// TwinCAT 3 PLC project TC_Sample
// ProgramVersion: 3.1.4023.0
// libraries:
//   Tc2_ControllerToolbox, * (Beckhoff Automation GmbH)
//   Tc2_Standard, * (Beckhoff Automation GmbH)
//   Tc2_System, * (Beckhoff Automation GmbH)
//   Tc2_TempController, * (Beckhoff Automation GmbH)
//   Tc3_Module, * (Beckhoff Automation GmbH)
//   VisuDialogs, * (System)
//   VisuSymbols,3.5.10.0,System
// project tree:
//   / GlobalTextList.TcGTLO, PlcTask.TcTTO, Visualization Manager.TcVMO
//   GVLs/ Scope_Variables.TcGVL
//   POUs/Controller/ Controller_v2.TcPOU
//   POUs/ MAIN.TcPOU
//   VISUs/ Visualization.TcVIS
// real-time tasks:
//   TASK PlcTask: cycle T#10ms, priority 20, ADS port 350
// I/O:
//   DEVICE Device 1 (EtherCAT), AmsNetId 5.47.60.12.2.1
//     Term 1 (EK1200) [EK1200-5000 EtherCAT Power supply (2A E-Bus)]
//       Term 2 (EL3204) [EL3204 4Ch. Ana. Input PT100 (RTD)]
//       Term 3 (EL2004) [EL2004 4Ch. Dig. Output 24V, 0.5A]
//       Term 4 (EL9011) [EL9011 End Terminal]
// variable links:
//   TC_Sample/TC_Sample Instance <-> Device 1 (EtherCAT)/Term 1 (EK1200)/Term 2 (EL3204)
//     PlcTask Inputs/Controller_v2.iTempre <-> RTD Inputs Channel 1/Value
//   TC_Sample/TC_Sample Instance <-> Device 1 (EtherCAT)/Term 1 (EK1200)/Term 3 (EL2004)
//     PlcTask Outputs/Controller_v2.bYPWMPos <-> Channel 1/Output

CONFIGURATION TC_Sample
    RESOURCE PLC ON TwinCAT3
        TASK PlcTask(INTERVAL := T#10ms, PRIORITY := 20);
        PROGRAM MAIN WITH PlcTask : MAIN;
    END_RESOURCE
END_CONFIGURATION

// ---- GVLs/Scope_Variables.TcGVL
VAR_GLOBAL
	fX_Scope	: LREAL;
	fY_Scope	: LREAL;
	fW_Scope	: LREAL;
END_VAR

// ---- POUs/MAIN.TcPOU
PROGRAM MAIN

VAR	
(* 选择功能块，温度控制库有两个功能块版本 V1和 V2 ，系统通过默认选择 V1，V1为旧版本，已被淘汰 *)
	nSelectController	: UINT := 1;	
	
(* 激活系统触发条件 *)	
	bStart				: BOOL;			
END_VAR

(* 调用功能块V2，需将nSelectController从1切换为2 *)
IF bStart THEN
	       	nSelectController:= 2  ;   
			Controller_v2();		
END_IF;

END_PROGRAM

// ---- POUs/Controller/Controller_v2.TcPOU
PROGRAM Controller_v2

VAR
	
		eCTRL_Mode 				: E_CTRL_MODE := eCTRL_MODE_Tune; 	(*控制模式*)
		bSelSetpoint			: BOOL	:= FALSE;
		
			iTempre AT %I*:INT;                                  (* 传输回未被转换的温度值 *)
			ftemp:LREAL;                                         (* 被转换的实际温度值 *)
		
		fW						: LREAL;						(* 设定值 *)
		fW1						: LREAL := 65.0;				(* 主设定值*)
		fW2						: LREAL := 45.0;				(* 辅助设定值*)		
		fY						: LREAL;						(* 模拟量输出中间变量 *)
		fX						: LREAL;						(* 设备真实的温度值 *)
		bYPWMPos				AT %Q*: BOOL;                   (* PWM输出，加热 *)
		bYPWMNeg				AT %Q*: BOOL;                   (* PWM输出，冷却 *)
		
		bNoise					: BOOL;                         (* 系统中是否存在错误 *)
		bError 					: BOOL;                         (* 存在错误的话，会生成一个错误代码 *)
		eErrorId 				: E_CTRL_ErrorCodes;
		
		stControllerParameter	: ST_CTRL_TempCtrlParameter := (		
		
		(*内部结构体参数 *)
		iMode					:= 1,											(*运作模式 ： 1=加热, 2=冷却, 3=加热以及冷却 *)
		iReactionOnFailure		:= eCTRL_ReactionOnFailure_StopController,		(*当系统产生错误时，系统反应： 0=关闭系统, 1=手动操作 *)
	
		bSelCtrlParameterSet	:= FALSE,										(* FALSE = 内部pid设定, TRUE = 外部pid设定 *)
	
		dwAlarmSupp				:= 16#0000EFFF,									(* 报警限制值 *)
		tCtrlCycleTime			:= T#500MS,										(* 控制器周期时间 *)
		tTaskCycleTime			:= T#10MS,										(* PLC任务周期时间 *)
		
		(*整定参数*)
		iTuningMode				:= 1,											(* 只加热、只冷却、先加热后冷却、先冷却后加热 *)
	
		tTuneStabilisation		:= T#5S,										(* 等待系统稳定下的时间 *)
	
		fEndTunePercentHeating	:= 80.0,										(* 大于80%，切换成闭环控制 *)
		fYTuneHeating			:= 100.0,										(* 加热协调操作时的阶跃变换 *)
		fYStableHeating			:= 0.0,											(* 加热调整操作 *)
	
		fEndTunePercentCooling	:= 20.0,										(* 小于20%，切换成闭环控制 *)
		fYTuneCooling			:= 0.0,									        (*冷却协调操作时的阶跃变换 *)
		fYStableCooling			:= 0.0,											(* 冷却调整操作 *)
		fScalingFactor			:= 1.0,											(*加热和冷却的KP比例系数 *)
		
		(*设定点参数*)
		fWMin					:= 0.0,											(*设定点的最小值 *)
		fWMax					:= 80.0,										(*设定点的最大值 *)
	
		(*软启动*)
		bEnableSoftStart		:= TRUE,										(* 启动方式：FALSE = 硬启动, TRUE = 软启动 *)
		bEnableRamping			:= FALSE,										(* 波形：FALSE = 无斜波, TRUE = 有斜波 *)
	
		fWStartUp				:= 55.0,										(* 软启动的预设定值 *)
		tStartUp				:= T#30S,										(* 软启动的等待时间*)
		bStartUpRamping			:= FALSE,										(* 启动过程时是否加入斜波 *)
		fWStartUpVeloPos		:= 0.3,											(* 启动过程时增加给定的最大梯度值*)
		fWStartUpVeloNeg		:= 0.3,											(* 启动过程时减小给定的最大梯度值 *)
	
		fWVeloPos				:= 0.5,											(* 增加给定的最大梯度值 *)
		fWVeloNeg				:= 0.5,											(* 减小给定的最大梯度值 *)	
	
		(* 实际值参数*)
		bFilter 				:= FALSE,                                       (* 是否启动实际值过滤器*)
		tFilter					:= T#0S,                                        (* 实际值过滤器的时间常数*)
		
		(* 死区参数 *)
		bDeadband				:= FALSE,                                       (* 是否加入死区 *)
		fEDeadband				:= 0.0,											(* 死区参数 *)
		
		(* 控制值参数*)
		fYMin					:= 0.0,											(* 控制器下限值 *)
		fYMax					:= 100.0,										(* 控制器上限值 *)
		fYManual				:= 0.0,									 		(* 手动操作值*)
		fYOnFailure				:= 0.0,											(* 故障时的手动控制值 *)
		tPWMCycleTime			:= T#1S,										(* PWM周期 *)
		tPWMMinOffTime			:= T#0S,										(* PWM最小的关闭时间*)
		tPWMMinOnTime			:= T#0S,										(* PWM最小的开启时间 *)
		tPWMWaitingTime			:= T#0S,										(* PWM从加热到冷却的切换时间*)
		tPWMCycleTimeCool       := T#1S,                                        (* PWM冷却周期 *)
	
		fYThresholdOff			:= 0.0,											(* 三步关闭极限，此例程不需要使用 *)
		fYThresholdOn			:= 0.0,											(* 三步开启极限，此例程不需要使用 *)
	
		nCyclesForSwitchOver	:= 100,                                         (* 参数级转换数 *) 
	
		(* 控制器设定 *)
		bEnablePreController 	:= FALSE,										(* 允许预控制器 *)
		bEnableZones 			:= FALSE,										(* 允许开环调节时的设定调节带 *)
		bEnableCVFilter 		:= FALSE,										(* 允许CV滤波 *)
		iFilterType 			:= 1,			 			                    (* CV滤波器类型，系统默认设定 *)
		iControllerType 		:= eCTRL_ControllerType_PID,					(* 控制器的PID类型，系统默认设定 *)
		
		
		(* 最小最大温度 *) 
		TempLow					:= -5.0,                                        (* 第一道报警值下限 *) 
		TempLowLow				:= -10.0,                                       (* 第二道报警值下限 *)
		TempHigh				:= 80.0,                                        (* 第一道报警值上限 *)
		TempHighHigh			:= 100.0,                                       (* 第二道报警值上限 *)
		TempAbsoluteHigh		:= 300.0,                                       (* 设定报警值上限 *)
		TempAbsoluteLow			:= 0.0,	                                        (* 设定报警值下限 *)
		
		(* 内部整定高级参数 *)
		fTuneKp					:= 1.0,                                         (* 比例 *)
		fTuneTn					:= 2.5,                                         (* 积分时间常数 *)
		fTuneTv					:= 0.42,                                        (* 微分时间常数 *)
		fTuneTd					:= 0.25                                         (* 阻尼时间常数 *)
		);
	
	fbTempController			: FB_CTRL_TempController;                       (* 功能块声明 *)
	

	fbCtrlParameter				: FB_CTRL_CtrlParameter;                        (* 功能块声明 *)
	stController				: ST_CTRL_ParaController;                       (* 结构体变量声明 *)
	 

	
END_VAR

(* 接收的温度数据转换 *)
ftemp:=INT_TO_LREAL (iTempre);
ftemp:=ftemp/10;
(* 选择设定点 *)
IF bSelSetpoint THEN
	fW := fW2;
ELSE
	fW := fW1;
END_IF


(* 实际温度值中间变量转换*)				
fbTempController.fX:=ftemp;		

(* 设置功能块参数，只需修改 fX:=ftemp *)
fbTempController(
					eCtrlMode				:= eCTRL_Mode, 
					bSelSetpoint			:= bSelSetpoint, 
					fW1						:= fW1, 
					fW2						:= fW2, 
					fX						:= ftemp, 
					fYManual				:= , 
					bOpenThermocouple		:= FALSE, 
					bReverseThermocouple	:= FALSE, 
					bBackVoltage			:= FALSE, 
					bLeakage				:= FALSE, 
					bShortCircuit			:= FALSE, 
					bOpenCircuit			:= FALSE, 
					sParaControllerExternal	:= stController, 
					sControllerParameter	:= stControllerParameter, 
					);
					 
(* 模拟量输出，此例程无需使用 *)			
//fY := fbTempController.fYAnalog;

(* PWM加热输出 *)
bYPWMPos := fbTempController.bYPWMPos;

(* PWM冷却输出，此例程无需使用 *)
//bYPWMNeg := fbTempController.bYPWMNeg;

bError := fbTempController.bError;
eErrorId := fbTempController.eErrorId;

(* 选择控制器模式。第一次使用时，eCTRL_Mode必须先进入自整定模式：eCTRL_STATE_TUNED 进行参数整定的操作*)
(* 参数整定之后，再进入主动模式使系统控制温度 *)
IF fbTempController.eCtrlState = eCTRL_STATE_TUNED THEN
	eCTRL_Mode := eCTRL_MODE_ACTIVE;	
END_IF

END_PROGRAM

// ---- GlobalTextList.TcGTLO
TEXTLIST GlobalTextList
  600 = '%.1f'
  720 = '%.2f'
  18 = '%1.f'
  575 = '%b'
  275 = '%d'
  993 = '%s'
  508 = '/'
  767 = 'Kp：'
  966 = 'PID参数设置'
  344 = 'PID参数设置：'
  965 = 'PWM脉冲信号：'
  173 = 'Td：'
  697 = 'Tn:'
  356 = 'Tn：'
  250 = 'Tv：'
  650 = '保温模式'
  83 = '保温模式温度(℃)：'
  706 = '保温模式温度数值：'
  919 = '保温模式温度：'
  821 = '关闭系统'
  324 = '加热(冷却)模式温度：'
  543 = '加热模式'
  123 = '加热（冷却）模式'
  224 = '启动程序'
  14 = '启动风扇'
  332 = '实际温度数值(℃)：'
  582 = '实际温度数值PWM脉冲信号：'
  410 = '实际温度数值：'
  909 = '开启（禁用）软启动'
  160 = '手动复位（后缀改为RESET）'
  629 = '手动复位（需将后缀改为RESET）'
  684 = '激活/关闭系统'
  418 = '激活系统'
  142 = '系统是否存在错误：'
  719 = '紧急停止按钮'
  730 = '自动化温度控制系统'
  338 = '设定温度(℃)：'
  804 = '设定温度：'
  6 = '软启动时间(ms)：'
  386 = '软启动时间（）ms：'
  976 = '软启动时间：'
  824 = '软启动温度(℃)：'
  92 = '软启动温度：'
  71 = '软启动设置'
  204 = '软启动设置：'
  682 = '错误代码'
  839 = '错误代码：'
END_TEXTLIST

// ---- VISUs/Visualization.TcVIS
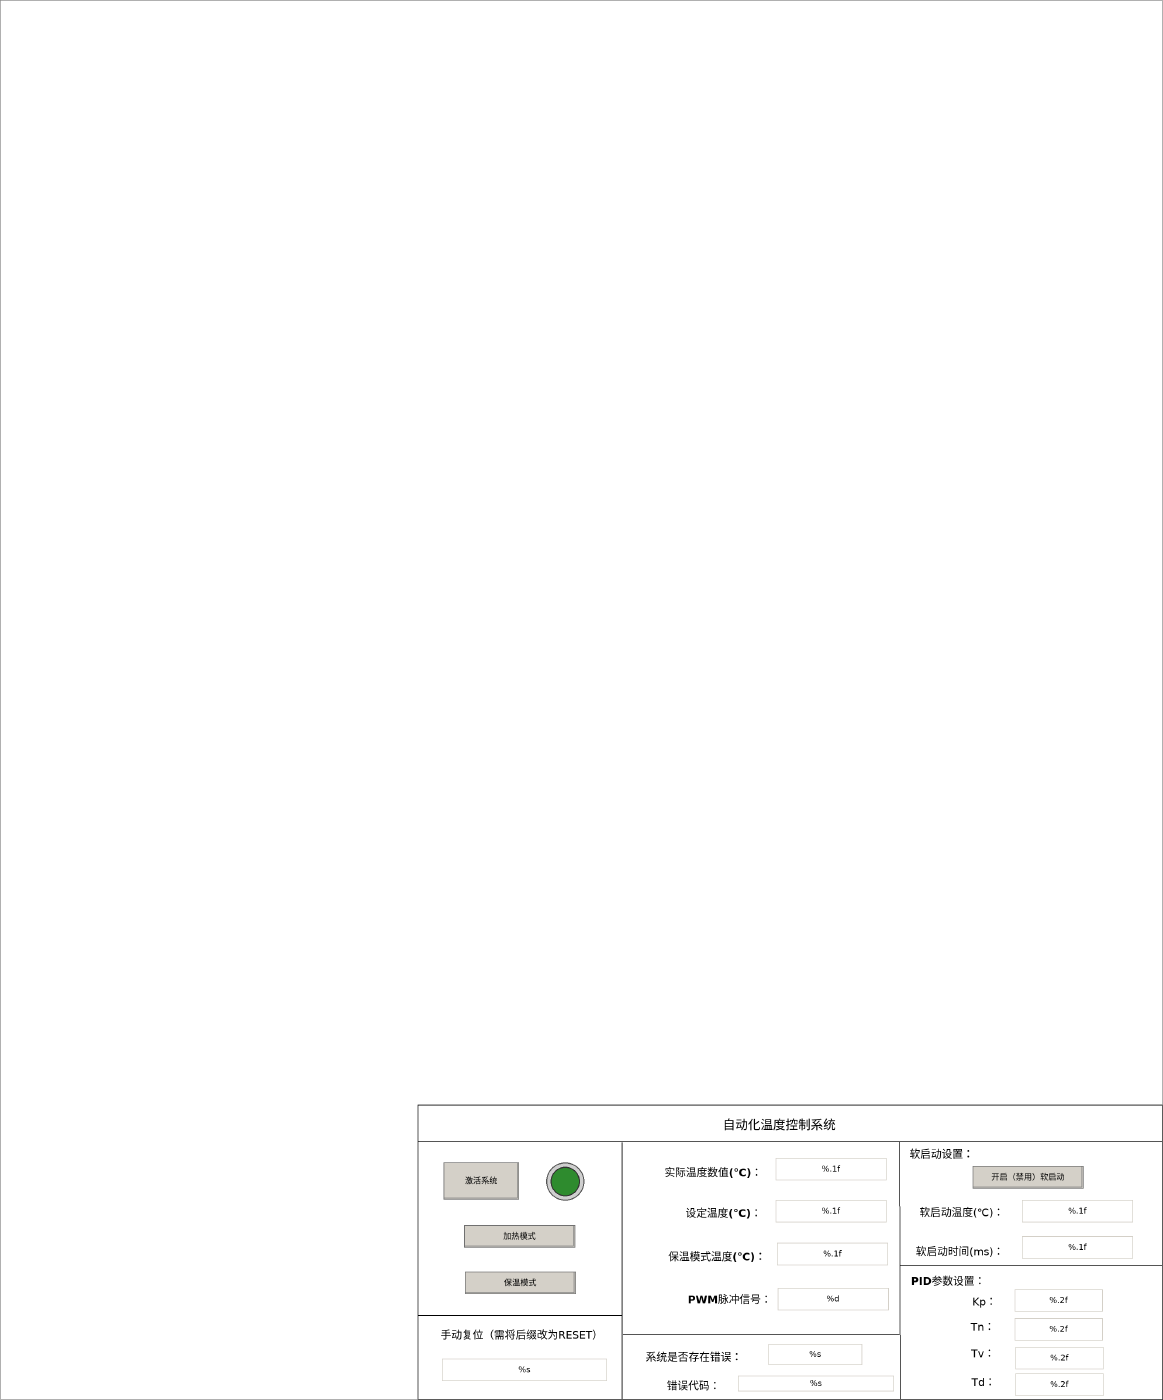
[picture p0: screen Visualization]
VISUALIZATION Visualization  // 1576x1897
    Rectangle (566,1497 1010x400)
    Line (1576,1547) (567,1547)
    Label (910,1502 292x44), "自动化温度控制系统"
    Button (601,1575 102x50), "激活系统"
        toggle MAIN.bStart p2164770859=TRUE
    Line (843,1897) (843,1548)
    Lamp1 (736,1570 60x62), variable: MAIN.bStart, style: Lamp-Lamp1-Green
    Button (629,1660 150x30), "加热模式"
        toggle Controller_v2.bSelSetpoint p2164770859=TRUE
    Button (630,1723 150x30), "保温模式"
        toggle Controller_v2.bSelSetpoint p2164770859=TRUE
    Textfield (1051,1569 150x30), "%.1f", text variable: Controller_v2.ftemp
    Textfield (1051,1626 150x30), "%.1f", text variable: Controller_v2.fW1
        OnMouseClick: write the text variable via Default
    Textfield (1053,1684 150x30), "%.1f", text variable: Controller_v2.fW2
        OnMouseClick: write the text variable via Default
    Textfield (1054,1745 150x30), "%d", text variable: Controller_v2.bYPWMPos
    Label (891,1570 151x38), "实际温度数值(℃)："
    Label (917,1626 127x36), "设定温度(℃)："
    Label (898,1685 147x36), "保温模式温度(℃)："
    Label (929,1743 120x36), "PWM脉冲信号："
    Line (1218,1808) (844,1808)
    Label (858,1826 165x26), "系统是否存在错误："
    Label (865,1863 150x30), "错误代码："
    Textfield (1000,1864 211x21), "%s", text variable: Controller_v2.eErrorId
    Textfield (1041,1821 127x28), "%s", text variable: Controller_v2.bError
    Textfield (599,1841 223x30), "%s", text variable: Controller_v2.eCTRL_Mode
        OnMouseClick: write the text variable via Default
    Label (579,1796 256x26), "手动复位（需将后缀改为RESET）"
    Line (567,1782) (842,1782)
    Line (1234,1549)
    Line (1220,1896) (1219,1547)
    Button (1318,1580 150x30), "开启（禁用）软启动"
        toggle Controller_v2.stControllerParameter.bEnableSoftStart p2164770859=TRUE
    Line (1575,1715) (1220,1715)
    Label (1213,1546 126x36), "软启动设置："
    Label (1235,1625 137x36), "软启动温度(℃)："
    Label (1231,1678 140x36), "软启动时间(ms)："
    Textfield (1385,1626 150x30), "%.1f", text variable: Controller_v2.stControllerParameter.fWStartUp
        OnMouseClick: write the text variable via Default
    Textfield (1385,1675 150x30), "%.1f", text variable: Controller_v2.stControllerParameter.tStartUp
        OnMouseClick: write the text variable via Default
    Label (1222,1718 126x36), "PID参数设置："
    Label (1271,1746 126x36), "Kp："
    Label (1269,1780 126x36), "Tn："
    Label (1269,1816 126x36), "Tv："
    Label (1270,1855 126x36), "Td："
    Textfield (1375,1747 119x30), "%.2f", text variable: Controller_v2.stControllerParameter.fTuneKp
        OnMouseClick: write the text variable via Default
    Textfield (1375,1786 119x30), "%.2f", text variable: Controller_v2.stControllerParameter.fTuneTn
        OnMouseClick: write the text variable via Default
    Textfield (1376,1825 119x30), "%.2f", text variable: Controller_v2.stControllerParameter.fTuneTv
        OnMouseClick: write the text variable via Default
    Textfield (1376,1861 119x30), "%.2f", text variable: Controller_v2.stControllerParameter.fTuneTd
        OnMouseClick: write the text variable via Default
END_VISUALIZATION
